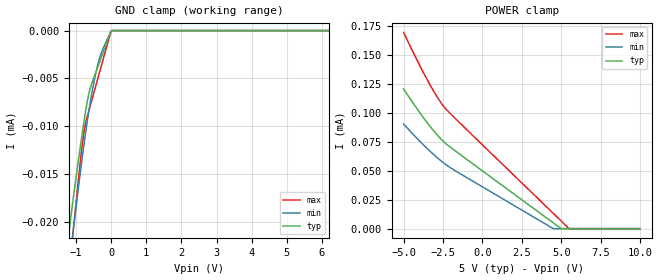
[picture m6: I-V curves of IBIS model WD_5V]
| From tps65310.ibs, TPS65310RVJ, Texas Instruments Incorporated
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[Model]   WD_5V
Model_type   Input
Vinl = .8
Vinh = 2.
|   typ   min   max
C_comp   0.01p   0.01p   0.01p
[Voltage Range]   5   4.5   5.5
[Temperature Range]   27   175   -40
[Power Clamp Reference]   5   4.5   5.5
[GND Clamp Reference]   -0   -0   -0
[GND Clamp]
|   Voltage   I(typ)   I(min)   I(max)
-5V       -190.4uA   -154.1uA   -253.9uA
-1.25V    -22.68uA   -26.35uA   -27.16uA
-1.16V    -19.81uA   -23.47uA   -23.81uA
-1.04V    -16.42uA   -19.71uA   -19.41uA
-800mV    -10.16uA   -12.62uA   -11.28uA
-740mV    -8.718uA   -11uA      -9.885uA
-650mV    -6.847uA   -8.749uA   -8.577uA
-500mV    -5.005uA   -5.56uA    -6.596uA
-380mV    -3.802uA   -3.54uA    -5.012uA
-290mV    -2.901uA   -2.437uA   -3.825uA
-5mV      -48.65nA   -38.7nA    -64.61nA
9.985V    0A         0A         0A
[POWER Clamp]
|   Voltage   I(typ)   I(min)   I(max)
-5V       120.9uA    90.54uA    169.8uA
-4.34V    107.6uA    80.88uA    151.2uA
-3.365V   89.33uA    67.59uA    125.5uA
-2.81V    80.23uA    60.8uA     112.7uA
-2.315V   73.52uA    55.44uA    103.5uA
4.495V    5.053uA    38.68nA    13.26uA
4.99V     98.39nA    0A         6.728uA
5.485V    0A         0A         196.4nA
9.985V    0A         0A         0A
